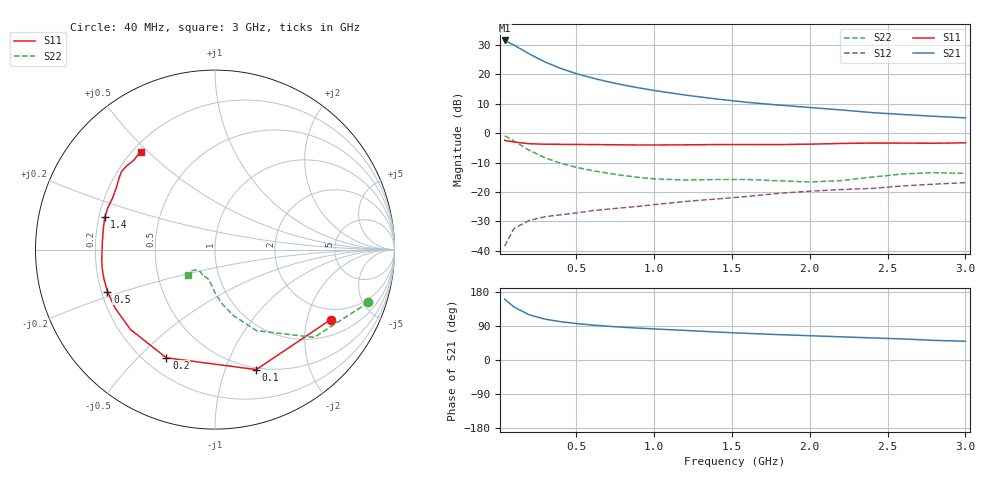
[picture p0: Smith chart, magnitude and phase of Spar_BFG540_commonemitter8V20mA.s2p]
! Filename:  BFG540I.S2P  Version:  3.0
! NXP part #: BFG540  Date: Feb 1992
! Bias condition: Vce=8V, Ic=20mA
! IN LINE PINNING: same data as with cross emitter pinning.
#  MHz  S  MA  R  50
! Freq  S11  S21  S12  S22  !GUM [dB]
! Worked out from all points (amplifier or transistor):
!   21 points, 40 MHz to 3 GHz, reference 50 ohm
!   highest |S21| = 31.5 dB at 40 MHz (marker M1)
!   |S21| within 3 dB of that: start of sweep to 146.8 MHz
!   unconditionally stable (mu >= 1): 954.4 MHz to end of sweep
!   at 300 MHz: K = 0.46, MSG = 26.3 dB, |S12| = -28.4 dB
!   at 1 GHz: K = 1.02, MAG = 18.6 dB, |S12| = -24.3 dB
!   at 3 GHz: K = 1.17, MAG = 8.5 dB, |S12| = -16.8 dB
!   lowest NFmin = 1.50 dB at 900 MHz
!   S11 on the Smith chart (normalised r, x): 40 MHz: 1.56, -2.81; 100 MHz: 0.48, -1.29; 200 MHz: 0.28, -0.61; 500 MHz: 0.22, -0.18; 1.4 GHz: 0.22, +0.14; 3 GHz: 0.23, +0.47
40  0.754 -31.1  37.62 160.6  0.012 73.4  0.904 -19.0
100  0.707 -71.0  31.38 140.0  0.024 57.2  0.738 -41.5
200  0.661 -114.2  22.11 118.9  0.033 45.2  0.508 -62.8
300  0.648 -136.6  16.19 107.9  0.038 42.1  0.381 -74.5
400  0.645 -149.9  12.61 101.1  0.041 42.1  0.308 -82.0
500  0.643 -158.7  10.29 96.2  0.044 43.2  0.263 -87.2
600  0.64 -165.4  8.698 92.4  0.048 45.4  0.232 -91.0
700  0.637 -170.7  7.518 89.2  0.051 47.5  0.209 -94.0
800  0.633 -175.4  6.617 86.5  0.054 49.3  0.191 -96.9
900  0.629 -179.8  5.894 84.1  0.057 51.4  0.177 -100.1
1000  0.629 176.1  5.32 82.0  0.061 53.3  0.167 -103.6
1200  0.633 169.3  4.445 78.0  0.069 55.7  0.16 -110.5
1400  0.64 163.7  3.812 73.9  0.076 57.2  0.163 -114.5
1600  0.641 158.8  3.338 70.2  0.084 59.7  0.163 -115.7
1800  0.639 153.2  3.004 67.0  0.095 60.0  0.155 -117.3
2000  0.65 147.5  2.73 64.1  0.103 61.4  0.148 -124.0
2200  0.668 143.0  2.482 61.1  0.11 61.9  0.156 -133.5
2400  0.679 139.9  2.236 58.3  0.115 62.9  0.179 -138.6
2600  0.678 136.7  2.073 55.6  0.127 62.4  0.203 -138.4
2800  0.673 132.4  1.935 51.8  0.136 60.5  0.213 -136.3
3000  0.685 127.2  1.818 49.5  0.144 61.3  0.207 -137.7
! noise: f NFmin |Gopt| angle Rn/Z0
900  1.5  0.232  140  0.14
2000  2.2  0.49  -163  0.11
